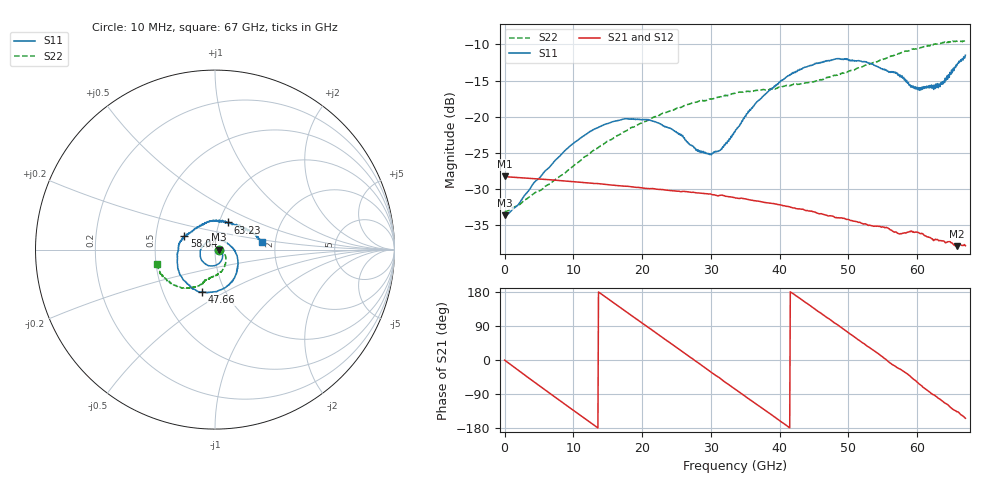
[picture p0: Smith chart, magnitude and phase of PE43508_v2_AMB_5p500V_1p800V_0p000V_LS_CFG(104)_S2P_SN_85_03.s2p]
!Keysight Technologies,N5227A,US51270237,A.10.43.00
!Date: Wednesday, August 22, 2018 17:17:32
!Correction: S11(Full 2 Port(1,3))
!S31(Full 2 Port(1,3))
!S13(Full 2 Port(1,3))
!S33(Full 2 Port(1,3))
!S2P File: Measurements: S11, S31, S13, S33:
# Hz S  dB  R 50
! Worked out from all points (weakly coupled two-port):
!   801 points, 10 MHz to 67 GHz, reference 50 ohm
!   highest |S21| = -28.29 dB at 10 MHz (marker M1); lowest = -37.9 dB at 65.74 GHz (marker M2)
!   lowest |S11| = -33.7 dB at 93.74 MHz (marker M3), VSWR 1.04, Z = 52.1 + j0.00331 ohm
!   |S11| at or under -10 dB: start of sweep to end of sweep
!   |S22| runs from -33.2 to -9.5 dB; largest |S21 - S12| = 0.0002
!   S11 on the Smith chart (normalised r, x): 10 MHz: 1.04, -0.00; 47.66 GHz: 0.78, -0.39; 58.04 GHz: 0.70, +0.11; 63.23 GHz: 1.10, +0.34; 67 GHz: 1.71, +0.15
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1e7  -33.62 -0.9  -28.29 -0.3  -28.31 -0.2  -33.14 -0.5
9.37375e7  -33.70 0.1  -28.32 -1.4  -28.33 -1.4  -33.17 0.3
1.935962e9  -32.23 0.2  -28.44 -26.4  -28.44 -26.4  -32.35 2.5
5.787888e9  -27.66 -18.9  -28.69 -77.5  -28.69 -77.5  -29.78 -1.4
1.123082e10  -22.83 -62.1  -29.10 -148.8  -29.11 -148.8  -25.90 -17.5
1.74274e10  -20.33 -111.7  -29.62 130.8  -29.62 130.8  -22.07 -39.2
2.236791e10  -20.88 -154.5  -30.08 67.0  -30.08 66.9  -19.87 -56.6
2.580115e10  -22.69 168.4  -30.37 23.1  -30.36 23.1  -18.65 -67.4
2.973681e10  -25.20 97.4  -30.72 -28.0  -30.72 -28.0  -17.58 -78.3
3.132782e10  -24.68 64.1  -30.91 -48.1  -30.91 -48.1  -17.25 -82.7
3.3505e10  -22.12 24.4  -31.24 -76.9  -31.25 -76.9  -16.77 -88.4
3.836178e10  -16.52 -30.8  -31.97 -138.8  -31.98 -138.8  -16.29 -97.4
4.162754e10  -14.14 -58.8  -32.57 178.9  -32.55 179.1  -15.70 -101.8
4.472582e10  -12.88 -83.6  -33.14 139.5  -33.11 139.5  -15.22 -105.6
4.765664e10  -12.14 -106.5  -33.78 102.0  -33.76 101.9  -14.39 -109.4
5.234594e10  -12.37 -143.9  -34.87 41.8  -34.84 41.7  -12.93 -115.2
5.586291e10  -13.86 -179.4  -35.52 -5.2  -35.49 -5.6  -11.72 -124.2
5.804009e10  -14.56 155.5  -36.13 -30.1  -36.14 -30.6  -10.99 -130.7
6.004979e10  -15.95 122.3  -36.01 -59.3  -36.03 -59.7  -10.59 -137.4
6.323181e10  -15.52 64.4  -37.17 -102.5  -37.21 -103.1  -9.90 -149.9
6.574394e10  -12.94 23.9  -37.95 -136.4  -38.04 -136.5  -9.56 -159.4
6.7e10  -11.50 8.7  -37.89 -153.7  -37.98 -153.9  -9.48 -165.8
